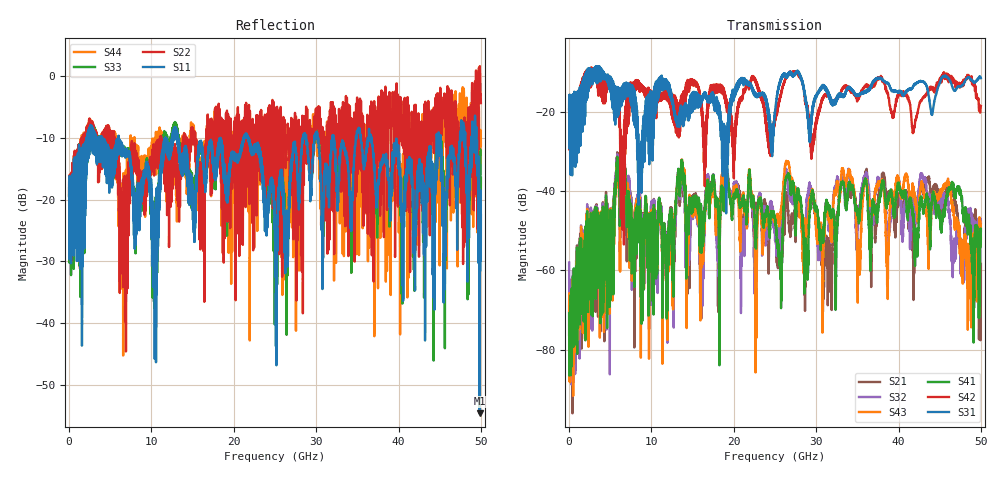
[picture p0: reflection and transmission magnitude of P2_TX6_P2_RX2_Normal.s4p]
!Keysight Technologies,N5225B,MY57041031,A.13.20.10
!Date: Friday, May 31, 2019 11:29:33
!Correction: S11(Full 4 Port(1,2,3,4))
!S12(Full 4 Port(1,2,3,4))
!S13(Full 4 Port(1,2,3,4))
!S14(Full 4 Port(1,2,3,4))
!S21(Full 4 Port(1,2,3,4))
!S22(Full 4 Port(1,2,3,4))
!S23(Full 4 Port(1,2,3,4))
!S24(Full 4 Port(1,2,3,4))
!S31(Full 4 Port(1,2,3,4))
!S32(Full 4 Port(1,2,3,4))
!S33(Full 4 Port(1,2,3,4))
!S34(Full 4 Port(1,2,3,4))
!S41(Full 4 Port(1,2,3,4))
!S42(Full 4 Port(1,2,3,4))
!S43(Full 4 Port(1,2,3,4))
!S44(Full 4 Port(1,2,3,4))
!S4P File: Measurements: <S11,S12,S13,S14>,
!<S21,S22,S23,S24>,
!<S31,S32,S33,S34>,
!<S41,S42,S43,S44>:
# Hz S  dB  R 50.0
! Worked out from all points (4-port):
!   5000 points, 10 MHz to 50 GHz, reference 50 ohm
!   strongest paths, dB at 10 MHz, 12.51 GHz, 25.01 GHz, 37.51 GHz, 50 GHz:
!     S31: -19.4, -16.8, -19.9, -11.6, -11.5
!     S42: -19.3, -15.9, -21.5, -11.2, -18.5
!     S41: -70.8, -48.5, -47.3, -43.4, -49.7
!     S43: -70.2, -50.9, -47.9, -38.6, -52.0
!     S32: -58.0, -49.1, -52.5, -36.7, -48.0
!     S21: -76.3, -46.3, -48.5, -42.3, -58.4
!   lowest |S11| = -54.6 dB at 49.84 GHz (marker M1), VSWR 1.00, Z = 50.2 + j0.0669 ohm
!   |S11| at or under -10 dB: 6.028 GHz to 11.67 GHz (5.641 GHz wide, 63.8 % of centre); 21.74 GHz to 28.38 GHz (6.639 GHz wide, 26.5 % of centre); 36.76 GHz to 44.63 GHz (7.867 GHz wide, 19.3 % of centre)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
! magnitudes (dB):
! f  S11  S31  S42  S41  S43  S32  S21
! 10 MHz  -19.4  -19.4  -19.3  -70.8  -70.2  -58.0  -76.3
! 6.58 GHz  -12.8  -14.9  -28.3  -32.0  -33.1  -31.5  -30.6
! 8.91 GHz  -17.2  -29.3  -13.7  -72.7  -55.3  -57.0  -49.2
! 13.77 GHz  -14.7  -19.8  -18.7  -34.0  -33.7  -34.8  -35.6
! 43.54 GHz  -13.0  -14.5  -15.1  -41.6  -48.7  -41.4  -36.5
! 49.84 GHz  -54.6  -11.1  -18.2  -61.0  -48.9  -48.5  -66.6
! 50 GHz  -22.5  -11.5  -18.5  -49.7  -52.0  -48.0  -58.4
